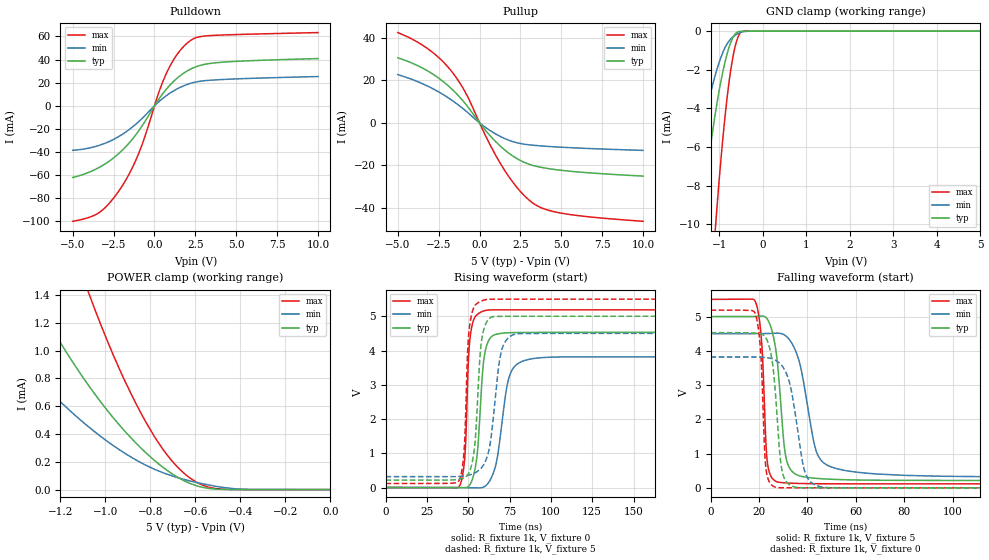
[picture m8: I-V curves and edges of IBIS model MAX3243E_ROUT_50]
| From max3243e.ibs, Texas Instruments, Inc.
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[Model]   MAX3243E_ROUT_50
Model_type  3-state
Enable   Active-High
Vref =   0
Rref =   3000
Cref =   150p
Vmeas =   1.5
| variable   typ   min   max
C_comp   3.21pF   2.84pF   3.64pF
| C_pullup   4.06pF   3.12pF   5.34pF
| C_pulldown   4.45pF   3.24pF   6.53pF
| C_tri-state   3.21pF   2.84pF   3.64pF
[Temperature Range]   40   100   -40
| Ambient temperature   25   85   -40
[Voltage range]   5   4.5   5.5
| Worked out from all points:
|   slope of the pulldown table from 0 to 0.75 V, typ, clamps not added: 50.5 ohm
|   slope of the pullup table from 0 to 0.75 V, typ, clamps not added: 108 ohm
|   GND clamp passes 1 mA (typ) near -0.80 V on its own axis
|   POWER clamp passes 1 mA (typ) near -1.18 V on its own axis
|   rising waveform, R_fixture 1k, V_fixture 0: 20-80 % time 3.89ns typ, 6.68ns min, 2.53ns max; typ from 0 V to 4.53 V
|   falling waveform, R_fixture 1k, V_fixture 5: 20-80 % time 3.58ns typ, 6.58ns min, 2.05ns max; typ from 5 V to 0.216 V
|   rising waveform, R_fixture 1k, V_fixture 5: 20-80 % time 3.68ns typ, 5.99ns min, 2.55ns max; typ from 0.216 V to 5 V
|   falling waveform, R_fixture 1k, V_fixture 0: 20-80 % time 3.12ns typ, 5.29ns min, 1.88ns max; typ from 4.53 V to 0 V
[GND Clamp]
| MAX3243E_ROUT_50
|   Voltage   I(typ)   I(min)   I(max)
-5V       -163.4mA   -113.4mA   -253.9mA
-1.73V    -17.53mA   -10.17mA   -35.95mA
-1.705V   -16.87mA   -9.761mA   -34.75mA
-1.405V   -9.813mA   -5.468mA   -21.46mA
-1.25V    -6.826mA   -3.717mA   -15.54mA
-1.08V    -4.109mA   -2.178mA   -9.935mA
-925mV    -2.174mA   -1.139mA   -5.731mA
-805mV    -1.056mA   -599.8uA   -3.16mA
-685mV    -316.1uA   -294.4uA   -1.315mA
-570mV    -32.22uA   -123.1uA   -306.2uA
-425mV    -293.2nA   -12.5uA    -3.703uA
5V        10.39pA    21.33uA    9.569pA
[POWER Clamp]
| MAX3243E_ROUT_50
|   Voltage   I(typ)   I(min)   I(max)
-5V       24.59mA    16.31mA    38.96mA
-1.625V   2.417mA    1.44mA     4.558mA
-1.59V    2.288mA    1.363mA    4.32mA
-1.315V   1.378mA    821.1uA    2.619mA
-1.195V   1.044mA    624.3uA    1.983mA
-1.075V   750.1uA    452.1uA    1.418mA
-935mV    459.3uA    283.6uA    857.8uA
-825mV    272.4uA    179.5uA    499.7uA
-725mV    137.7uA    110.4uA    248uA
-645mV    59.75uA    71.13uA    109.8uA
-510mV    3.805uA    24.04uA    7.633uA
-84.45fV  10.39pA    40.97pA    11.12pA
[Pulldown]
| MAX3243E_ROUT_50
|   Voltage   I(typ)   I(min)   I(max)
-5V       -61.93mA   -38.44mA   -99.84mA
-3.355V   -53.04mA   -34.05mA   -92.02mA
-2.015V   -38.98mA   -25.07mA   -70.14mA
-1.43V    -30.12mA   -19.2mA    -55.64mA
-910mV    -20.51mA   -12.91mA   -39.18mA
250mV     5.49mA     3.337mA    11.05mA
740mV     14.69mA    8.978mA    28.45mA
1.395V    24.09mA    14.78mA    44.71mA
2.11V     31.07mA    19.04mA    55.58mA
2.71V     34.64mA    21.1mA     59.64mA
3.92V     37.5mA     22.62mA    61.16mA
10V       40.91mA    25.36mA    63.4mA
[Pullup]
| MAX3243E_ROUT_50
|   Voltage   I(typ)   I(min)   I(max)
-5V       30.65mA    22.74mA    42.55mA
-3.125V   24.25mA    17.13mA    34.7mA
-2.355V   20.24mA    13.92mA    29.74mA
-1.685V   15.84mA    10.61mA    24.03mA
-815mV    8.508mA    5.458mA    13.62mA
470mV     -4.513mA   -2.725mA   -7.675mA
1.36V     -11.59mA   -6.761mA   -20.22mA
2.28V     -16.82mA   -9.362mA   -30.36mA
3.18V     -19.87mA   -10.47mA   -37.33mA
3.935V    -21.2mA    -10.96mA   -40.5mA
5.085V    -22.44mA   -11.51mA   -42.67mA
10V       -25.09mA   -12.97mA   -46.39mA
[Ramp]
| MAX3243E_ROUT_50
| variable   typ   min   max
dV/dt_r   2.72/3.90E-09   2.30/6.69E-09   3.12/2.53E-09
dV/dt_f   2.88/3.60E-09   2.52/6.59E-09   3.23/2.06E-09
R_load = 1k
[Rising Waveform]
| MAX3243E_ROUT_50
R_fixture =   1k
C_fixture =   0
L_fixture =   0
V_fixture =   0
V_fixture_min = 0
V_fixture_max = 0
|   Time   V(typ)   V(min)   V(max)
0s        591.1pV    1.593nV    266.5pV
44.9ns    -4.651mV   -1.979mV   62.45mV
48.1ns    -7.676mV   -3.454mV   992mV
51.3ns    103.3mV    -5.852mV   4.436V
55.4ns    948.1mV    -9.749mV   5.046V
58.6ns    3.306V     1.306mV    5.141V
63.9ns    4.397V     272.2mV    5.186V
74.5ns    4.519V     3.181V     5.187V
83.4ns    4.527V     3.698V     5.187V
269.9ns   4.528V     3.818V     5.187V
[Falling Waveform]
| MAX3243E_ROUT_50
R_fixture =   1k
C_fixture =   0
L_fixture =   0
V_fixture =   5
V_fixture_min = 4.5
V_fixture_max = 5.5
|   Time   V(typ)   V(min)   V(max)
0s        5V         4.5V       5.5V
18.7ns    5.004V     4.5V       5.401V
21.1ns    5.012V     4.502V     4.232V
23.4ns    4.927V     4.504V     772.9mV
27.7ns    3.575V     4.514V     171.4mV
30.4ns    1.225V     4.466V     147.5mV
32.5ns    594.3mV    4.329V     138.6mV
43.8ns    277.2mV    1.036V     121mV
52.8ns    242.8mV    546.4mV    118.2mV
269.9ns   216.3mV    317.4mV    117.2mV
[Rising Waveform]
| MAX3243E_ROUT_50
R_fixture =   1k
C_fixture =   0
L_fixture =   0
V_fixture =   5
V_fixture_min = 4.5
V_fixture_max = 5.5
|   Time   V(typ)   V(min)   V(max)
0s        216.3mV    317.4mV    117.2mV
44.6ns    241.9mV    325.3mV    217.9mV
47.6ns    284.4mV    339.7mV    1.128V
50.8ns    466.2mV    368.1mV    4.697V
54.1ns    1.303V     427.2mV    5.318V
58.1ns    4.293V     581.6mV    5.448V
63.1ns    4.947V     1.228V     5.498V
69.9ns    4.997V     3.943V     5.5V
77.3ns    4.999V     4.463V     5.5V
269.9ns   5V         4.5V       5.5V
[Falling Waveform]
| MAX3243E_ROUT_50
R_fixture =   1k
C_fixture =   0
L_fixture =   0
V_fixture =   0
V_fixture_min = 0
V_fixture_max = 0
|   Time   V(typ)   V(min)   V(max)
0s        4.528V     3.818V     5.187V
18.5ns    4.518V     3.819V     5.071V
20.7ns    4.493V     3.815V     3.933V
22.9ns    4.369V     3.804V     537.7mV
26.9ns    2.647V     3.721V     16.31mV
28.8ns    836.6mV    3.617V     2.84mV
30.6ns    259.1mV    3.441V     1.959mV
38.9ns    3.549mV    475.3mV    654uV
45.5ns    1.909mV    30.98mV    292.4uV
269.9ns   607.5pV    88.01nV    269.4pV
